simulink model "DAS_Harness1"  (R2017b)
settings: Solver=FixedStepDiscrete  StartTime=0.0  StopTime=1  FixedStep=0.01  RelTol=1e-3  EnableMultiTasking=on
undefined symbols (not defined in the file): sigbuilder_block
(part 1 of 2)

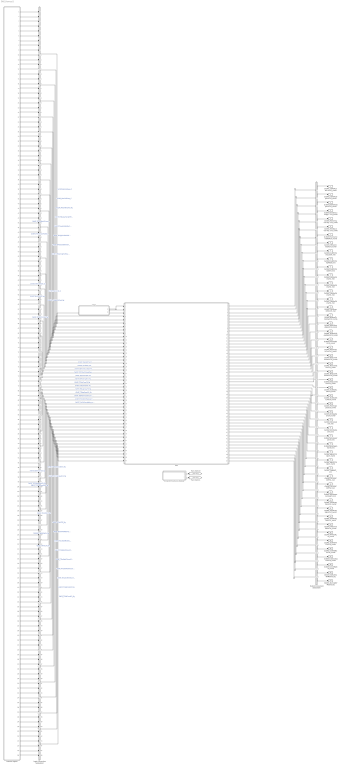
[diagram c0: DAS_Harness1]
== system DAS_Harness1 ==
  Chart : Stateflow chart  TreatAsAtomicUnit=on
  DAS : ModelReference  ModelNameDialog=DAS  SimulationMode=Normal  ModelReferenceVersion='M104C103'
  Harness Inputs : Subsystem  Tag=STV Subsys  LoadFcn=sigbuilder_block('load');  StartFcn=sigbuilder_block('start');  StopFcn=sigbuilder_block('stop');  ClipboardFcn=sigbuilder_block('clipboard');  mask(Sigbuilder block){tuvar=[0:10]}
      mask init:
      | if ~strcmp(get_param(bdroot(gcb),'SimulationStatus'),'stopped'),tuvar = sigbuilder_block('maskInit'); end
  Input Conversion Subsystem : Subsystem  Tag=__SLT_ICS__  Description=Signal spec. and routing
  Output Conversion Subsystem : Subsystem  Tag=__SLT_OCS__  Description=Signal spec. and routing
  Simulink Function scheduler : Test Sequence  Tag=__SLT_FCN_CALL__  TreatAsAtomicUnit=on
  GcDAS_CellVoltLowrLimCnt_numb : Outport  OutDataTypeStr=uint16  PortDimensions=[1]
  GcDAS_CellVoltUpprLimCnt_numb : Outport  Port=2  OutDataTypeStr=uint16  PortDimensions=[1]
  GcDAS_BattVoltUpprLimCnt_numb : Outport  Port=3  OutDataTypeStr=uint16  PortDimensions=[1]
  GcDAS_PackDisCurrUpprLimCnt_numb : Outport  Port=4  OutDataTypeStr=uint16  PortDimensions=[1]
  GcDAS_PackChrgCurrUpprLimCnt_numb : Outport  Port=5  OutDataTypeStr=uint16  PortDimensions=[1]
  GcDAS_FeedbackCurrUpprLimCnt_numb : Outport  Port=6  OutDataTypeStr=uint16  PortDimensions=[1]
  GcDAS_PackCurrLim500ACnt_numb : Outport  Port=7  OutDataTypeStr=uint32  PortDimensions=[1]
  GcDAS_TFPackCrntSafCnt_numb : Outport  Port=8  OutDataTypeStr=uint16  PortDimensions=[1]
  GcDAS_CellMinTempLowTi_min : Outport  Port=9  OutDataTypeStr=single  PortDimensions=[1]
  GcDAS_CellMinTempMidTi_min : Outport  Port=10  OutDataTypeStr=single  PortDimensions=[1]
  GcDAS_CellMinTempHiTi_min : Outport  Port=11  OutDataTypeStr=single  PortDimensions=[1]
  GcDAS_CellMaxTempTi1_min : Outport  Port=12  OutDataTypeStr=single  PortDimensions=[1]
  GcDAS_CellMaxTempTi2_min : Outport  Port=13  OutDataTypeStr=single  PortDimensions=[1]
  GcDAS_CellMaxTempTi3_min : Outport  Port=14  OutDataTypeStr=single  PortDimensions=[1]
  GcDAS_CellMaxTempTi4_min : Outport  Port=15  OutDataTypeStr=single  PortDimensions=[1]
  GcDAS_CellTempDiffLimTi_min : Outport  Port=16  OutDataTypeStr=single  PortDimensions=[1]
  GcDAS_BusbarTempHighCnt_numb : Outport  Port=17  OutDataTypeStr=uint16  PortDimensions=[1]
  GcDAS_PosCtlLoadOpenCnt_numb : Outport  Port=18  OutDataTypeStr=uint16  PortDimensions=[1]
  GcDAS_DCPosCtlLoadOpenCnt_numb : Outport  Port=19  OutDataTypeStr=uint16  PortDimensions=[1]
  GcDAS_PreChrgFailCnt_numb : Outport  Port=20  OutDataTypeStr=uint16  PortDimensions=[1]
  GcDAS_PreChrgOvrCurrCnt_numb : Outport  Port=21  OutDataTypeStr=uint16  PortDimensions=[1]
  GcDAS_PosContAdhesionCnt_numb : Outport  Port=22  OutDataTypeStr=uint16  PortDimensions=[1]
  GcDAS_PosContStuckCnt_numb : Outport  Port=23  OutDataTypeStr=uint16  PortDimensions=[1]
  GcDAS_NegContAdhesionCnt_numb : Outport  Port=24  OutDataTypeStr=uint16  PortDimensions=[1]
  GcDAS_NegContStuckCnt_numb : Outport  Port=25  OutDataTypeStr=uint16  PortDimensions=[1]
  GcDAS_KL30VoltLowCnt_numb : Outport  Port=26  OutDataTypeStr=uint16  PortDimensions=[1]
  GcDAS_KL30CVoltLowCnt_numb : Outport  Port=27  OutDataTypeStr=uint16  PortDimensions=[1]
  GcDAS_PreChrgOpenCnt_numb : Outport  Port=28  OutDataTypeStr=uint16  PortDimensions=[1]
  GcDAS_DCNegOpenCnt_numb : Outport  Port=29  OutDataTypeStr=uint16  PortDimensions=[1]
  GcDAS_SOCLowLimTi_min : Outport  Port=30  OutDataTypeStr=single  PortDimensions=[1]
  GcDAS_SOCHighLimTi_min : Outport  Port=31  OutDataTypeStr=single  PortDimensions=[1]
  GcDAS_SOHLowerLimTi_min : Outport  Port=32  OutDataTypeStr=single  PortDimensions=[1]
  GcDAS_BMSOperationTi_min : Outport  Port=33  OutDataTypeStr=single  PortDimensions=[1]
  GcDAS_BMSACChrgCnt_numb : Outport  Port=34  OutDataTypeStr=uint16  PortDimensions=[1]
  GcDAS_BMSDCChrgCnt_numb : Outport  Port=35  OutDataTypeStr=uint16  PortDimensions=[1]
  GcDAS_CellBalTi_min : Outport  Port=36  OutDataTypeStr=single  PortDimensions=[1]
  GcDAS_OCVSOCDiffTi1_min : Outport  Port=37  OutDataTypeStr=single  PortDimensions=[1]
  GcDAS_OCVSOCDiffTi2_min : Outport  Port=38  OutDataTypeStr=single  PortDimensions=[1]
  GcDAS_SOHLowerLimSaleTi_min : Outport  Port=39  OutDataTypeStr=single  PortDimensions=[1]
  GcDAS_ThmRnwyWarnCnt_numb : Outport  Port=40  OutDataTypeStr=uint16  PortDimensions=[1]
  GcDAS_ThmRnwyAlarmCnt_numb : Outport  Port=41  OutDataTypeStr=uint16  PortDimensions=[1]
  GcDAS_ThmRnwyFaultCnt_numb : Outport  Port=42  OutDataTypeStr=uint16  PortDimensions=[1]
  GcDAS_TPLEventWakeCnt_numb : Outport  Port=43  OutDataTypeStr=uint16  PortDimensions=[1]
  GcDAS_HVILFailCnt_numb : Outport  Port=44  OutDataTypeStr=uint16  PortDimensions=[1]
  GcDAS_IsoHVOFFChkCnt_numb : Outport  Port=45  OutDataTypeStr=uint16  PortDimensions=[1]
  GcDAS_IsoHVONChkCnt_numb : Outport  Port=46  OutDataTypeStr=uint16  PortDimensions=[1]
  GcDAS_IsoDCChrgChkCnt_numb : Outport  Port=47  OutDataTypeStr=uint16  PortDimensions=[1]
  GcDAS_CrashNplCnt_numb : Outport  Port=48  OutDataTypeStr=uint16  PortDimensions=[1]
  GbDAS_HVSafetyNVMStore_flg : Outport  Port=49  OutDataTypeStr=boolean  PortDimensions=[1]
  GbDAS_NormalNVMStore_flg : Outport  Port=50  OutDataTypeStr=boolean  PortDimensions=[1]
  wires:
  Harness Inputs/1(GcCDP_MinCellTemp_C) -> Input Conversion Subsystem/1(Inport_1)
  Harness Inputs/2(GcCDP_MaxCellTemp_C) -> Input Conversion Subsystem/2(Inport_2)
  Harness Inputs/3(GbCDP_AllCellTempVld_flg) -> Input Conversion Subsystem/3(Inport_3)
  Harness Inputs/4(GbISP_TFBusbarTempHiFltLv3_flg) -> Input Conversion Subsystem/4(Inport_4)
  Harness Inputs/5(GbISP_TFLowCellVoltSaf_flg) -> Input Conversion Subsystem/5(Inport_5)
  Harness Inputs/6(GbISP_TFHighCellVoltSaf_flg) -> Input Conversion Subsystem/6(Inport_6)
  Harness Inputs/7(GbISP_TFPackVoltHiAlrmFlt_flg) -> Input Conversion Subsystem/7(Inport_7)
  Harness Inputs/8(GbISP_TFDisChrgPwrFltLevel3_flg) -> Input Conversion Subsystem/8(Inport_8)
  Harness Inputs/9(GbISP_TFChrgPwrFltLevel3_flg) -> Input Conversion Subsystem/9(Inport_9)
  Harness Inputs/10(GbISP_TFFeedbackPwrFltLevel3_flg) -> Input Conversion Subsystem/10(Inport_10)
  Harness Inputs/11(GbISP_TFPackCrntSaf_flg) -> Input Conversion Subsystem/11(Inport_11)
  Harness Inputs/12(GcHDP_PackCrnt_A) -> Input Conversion Subsystem/12(Inport_12)
  Harness Inputs/13(GaCBC_CellBalCtlCmd_flg(1)) -> Input Conversion Subsystem/13(Inport_13)
  Harness Inputs/14(GaCBC_CellBalCtlCmd_flg(2)) -> Input Conversion Subsystem/14(Inport_14)
  Harness Inputs/15(GaCBC_CellBalCtlCmd_flg(3)) -> Input Conversion Subsystem/15(Inport_15)
  Harness Inputs/16(GaCBC_CellBalCtlCmd_flg(4)) -> Input Conversion Subsystem/16(Inport_16)
  Harness Inputs/17(GaCBC_CellBalCtlCmd_flg(5)) -> Input Conversion Subsystem/17(Inport_17)
  Harness Inputs/18(GaCBC_CellBalCtlCmd_flg(6)) -> Input Conversion Subsystem/18(Inport_18)
  Harness Inputs/19(GaCBC_CellBalCtlCmd_flg(7)) -> Input Conversion Subsystem/19(Inport_19)
  Harness Inputs/20(GaCBC_CellBalCtlCmd_flg(8)) -> Input Conversion Subsystem/20(Inport_20)
  Harness Inputs/21(GaCBC_CellBalCtlCmd_flg(9)) -> Input Conversion Subsystem/21(Inport_21)
  Harness Inputs/22(GaCBC_CellBalCtlCmd_flg(10)) -> Input Conversion Subsystem/22(Inport_22)
  Harness Inputs/23(GaCBC_CellBalCtlCmd_flg(11)) -> Input Conversion Subsystem/23(Inport_23)
  Harness Inputs/24(GaCBC_CellBalCtlCmd_flg(12)) -> Input Conversion Subsystem/24(Inport_24)
  Harness Inputs/25(GaCBC_CellBalCtlCmd_flg(13)) -> Input Conversion Subsystem/25(Inport_25)
  Harness Inputs/26(GaCBC_CellBalCtlCmd_flg(14)) -> Input Conversion Subsystem/26(Inport_26)
  Harness Inputs/27(GaCBC_CellBalCtlCmd_flg(15)) -> Input Conversion Subsystem/27(Inport_27)
  Harness Inputs/28(GaCBC_CellBalCtlCmd_flg(16)) -> Input Conversion Subsystem/28(Inport_28)
  Harness Inputs/29(GaCBC_CellBalCtlCmd_flg(17)) -> Input Conversion Subsystem/29(Inport_29)
  Harness Inputs/30(GaCBC_CellBalCtlCmd_flg(18)) -> Input Conversion Subsystem/30(Inport_30)
  Harness Inputs/31(GaCBC_CellBalCtlCmd_flg(19)) -> Input Conversion Subsystem/31(Inport_31)
  Harness Inputs/32(GaCBC_CellBalCtlCmd_flg(20)) -> Input Conversion Subsystem/32(Inport_32)
  Harness Inputs/33(GaCBC_CellBalCtlCmd_flg(21)) -> Input Conversion Subsystem/33(Inport_33)
  Harness Inputs/34(GaCBC_CellBalCtlCmd_flg(22)) -> Input Conversion Subsystem/34(Inport_34)
  Harness Inputs/35(GaCBC_CellBalCtlCmd_flg(23)) -> Input Conversion Subsystem/35(Inport_35)
  Harness Inputs/36(GaCBC_CellBalCtlCmd_flg(24)) -> Input Conversion Subsystem/36(Inport_36)
  Harness Inputs/37(GaCBC_CellBalCtlCmd_flg(25)) -> Input Conversion Subsystem/37(Inport_37)
  Harness Inputs/38(GaCBC_CellBalCtlCmd_flg(26)) -> Input Conversion Subsystem/38(Inport_38)
  Harness Inputs/39(GaCBC_CellBalCtlCmd_flg(27)) -> Input Conversion Subsystem/39(Inport_39)
  Harness Inputs/40(GaCBC_CellBalCtlCmd_flg(28)) -> Input Conversion Subsystem/40(Inport_40)
  Harness Inputs/41(GaCBC_CellBalCtlCmd_flg(29)) -> Input Conversion Subsystem/41(Inport_41)
  Harness Inputs/42(GaCBC_CellBalCtlCmd_flg(30)) -> Input Conversion Subsystem/42(Inport_42)
  Harness Inputs/43(GaCBC_CellBalCtlCmd_flg(31)) -> Input Conversion Subsystem/43(Inport_43)
  Harness Inputs/44(GaCBC_CellBalCtlCmd_flg(32)) -> Input Conversion Subsystem/44(Inport_44)
  Harness Inputs/45(GaCBC_CellBalCtlCmd_flg(33)) -> Input Conversion Subsystem/45(Inport_45)
  Harness Inputs/46(GaCBC_CellBalCtlCmd_flg(34)) -> Input Conversion Subsystem/46(Inport_46)
  Harness Inputs/47(GaCBC_CellBalCtlCmd_flg(35)) -> Input Conversion Subsystem/47(Inport_47)
  Harness Inputs/48(GaCBC_CellBalCtlCmd_flg(36)) -> Input Conversion Subsystem/48(Inport_48)
  Harness Inputs/49(GaCBC_CellBalCtlCmd_flg(37)) -> Input Conversion Subsystem/49(Inport_49)
  Harness Inputs/50(GaCBC_CellBalCtlCmd_flg(38)) -> Input Conversion Subsystem/50(Inport_50)
  Harness Inputs/51(GaCBC_CellBalCtlCmd_flg(39)) -> Input Conversion Subsystem/51(Inport_51)
  Harness Inputs/52(GaCBC_CellBalCtlCmd_flg(40)) -> Input Conversion Subsystem/52(Inport_52)
  Harness Inputs/53(GaCBC_CellBalCtlCmd_flg(41)) -> Input Conversion Subsystem/53(Inport_53)
  Harness Inputs/54(GaCBC_CellBalCtlCmd_flg(42)) -> Input Conversion Subsystem/54(Inport_54)
  Harness Inputs/55(GaCBC_CellBalCtlCmd_flg(43)) -> Input Conversion Subsystem/55(Inport_55)
  Harness Inputs/56(GaCBC_CellBalCtlCmd_flg(44)) -> Input Conversion Subsystem/56(Inport_56)
  Harness Inputs/57(GaCBC_CellBalCtlCmd_flg(45)) -> Input Conversion Subsystem/57(Inport_57)
  Harness Inputs/58(GaCBC_CellBalCtlCmd_flg(46)) -> Input Conversion Subsystem/58(Inport_58)
  Harness Inputs/59(GaCBC_CellBalCtlCmd_flg(47)) -> Input Conversion Subsystem/59(Inport_59)
  Harness Inputs/60(GaCBC_CellBalCtlCmd_flg(48)) -> Input Conversion Subsystem/60(Inport_60)
  Harness Inputs/61(GaCBC_CellBalCtlCmd_flg(49)) -> Input Conversion Subsystem/61(Inport_61)
  Harness Inputs/62(GaCBC_CellBalCtlCmd_flg(50)) -> Input Conversion Subsystem/62(Inport_62)
  Harness Inputs/63(GaCBC_CellBalCtlCmd_flg(51)) -> Input Conversion Subsystem/63(Inport_63)
  Harness Inputs/64(GaCBC_CellBalCtlCmd_flg(52)) -> Input Conversion Subsystem/64(Inport_64)
  Harness Inputs/65(GaCBC_CellBalCtlCmd_flg(53)) -> Input Conversion Subsystem/65(Inport_65)
  Harness Inputs/66(GaCBC_CellBalCtlCmd_flg(54)) -> Input Conversion Subsystem/66(Inport_66)
  Harness Inputs/67(GaCBC_CellBalCtlCmd_flg(55)) -> Input Conversion Subsystem/67(Inport_67)
  Harness Inputs/68(GaCBC_CellBalCtlCmd_flg(56)) -> Input Conversion Subsystem/68(Inport_68)
  Harness Inputs/69(GaCBC_CellBalCtlCmd_flg(57)) -> Input Conversion Subsystem/69(Inport_69)
  Harness Inputs/70(GaCBC_CellBalCtlCmd_flg(58)) -> Input Conversion Subsystem/70(Inport_70)
  Harness Inputs/71(GaCBC_CellBalCtlCmd_flg(59)) -> Input Conversion Subsystem/71(Inport_71)
  Harness Inputs/72(GaCBC_CellBalCtlCmd_flg(60)) -> Input Conversion Subsystem/72(Inport_72)
  Harness Inputs/73(GaCBC_CellBalCtlCmd_flg(61)) -> Input Conversion Subsystem/73(Inport_73)
  Harness Inputs/74(GaCBC_CellBalCtlCmd_flg(62)) -> Input Conversion Subsystem/74(Inport_74)
  Harness Inputs/75(GaCBC_CellBalCtlCmd_flg(63)) -> Input Conversion Subsystem/75(Inport_75)
  Harness Inputs/76(GaCBC_CellBalCtlCmd_flg(64)) -> Input Conversion Subsystem/76(Inport_76)
  Harness Inputs/77(GaCBC_CellBalCtlCmd_flg(65)) -> Input Conversion Subsystem/77(Inport_77)
  Harness Inputs/78(GaCBC_CellBalCtlCmd_flg(66)) -> Input Conversion Subsystem/78(Inport_78)
  Harness Inputs/79(GaCBC_CellBalCtlCmd_flg(67)) -> Input Conversion Subsystem/79(Inport_79)
  Harness Inputs/80(GaCBC_CellBalCtlCmd_flg(68)) -> Input Conversion Subsystem/80(Inport_80)
  Harness Inputs/81(GaCBC_CellBalCtlCmd_flg(69)) -> Input Conversion Subsystem/81(Inport_81)
  Harness Inputs/82(GaCBC_CellBalCtlCmd_flg(70)) -> Input Conversion Subsystem/82(Inport_82)
  Harness Inputs/83(GaCBC_CellBalCtlCmd_flg(71)) -> Input Conversion Subsystem/83(Inport_83)
  Harness Inputs/84(GaCBC_CellBalCtlCmd_flg(72)) -> Input Conversion Subsystem/84(Inport_84)
  Harness Inputs/85(GaCBC_CellBalCtlCmd_flg(73)) -> Input Conversion Subsystem/85(Inport_85)
  Harness Inputs/86(GaCBC_CellBalCtlCmd_flg(74)) -> Input Conversion Subsystem/86(Inport_86)
  Harness Inputs/87(GaCBC_CellBalCtlCmd_flg(75)) -> Input Conversion Subsystem/87(Inport_87)
  Harness Inputs/88(GaCBC_CellBalCtlCmd_flg(76)) -> Input Conversion Subsystem/88(Inport_88)
  Harness Inputs/89(GaCBC_CellBalCtlCmd_flg(77)) -> Input Conversion Subsystem/89(Inport_89)
  Harness Inputs/90(GaCBC_CellBalCtlCmd_flg(78)) -> Input Conversion Subsystem/90(Inport_90)
  Harness Inputs/91(GaCBC_CellBalCtlCmd_flg(79)) -> Input Conversion Subsystem/91(Inport_91)
  Harness Inputs/92(GaCBC_CellBalCtlCmd_flg(80)) -> Input Conversion Subsystem/92(Inport_92)
  Harness Inputs/93(GaCBC_CellBalCtlCmd_flg(81)) -> Input Conversion Subsystem/93(Inport_93)
  Harness Inputs/94(GaCBC_CellBalCtlCmd_flg(82)) -> Input Conversion Subsystem/94(Inport_94)
  Harness Inputs/95(GaCBC_CellBalCtlCmd_flg(83)) -> Input Conversion Subsystem/95(Inport_95)
  Harness Inputs/96(GaCBC_CellBalCtlCmd_flg(84)) -> Input Conversion Subsystem/96(Inport_96)
  Harness Inputs/97(GaCBC_CellBalCtlCmd_flg(85)) -> Input Conversion Subsystem/97(Inport_97)
  Harness Inputs/98(GaCBC_CellBalCtlCmd_flg(86)) -> Input Conversion Subsystem/98(Inport_98)
  Harness Inputs/99(GaCBC_CellBalCtlCmd_flg(87)) -> Input Conversion Subsystem/99(Inport_99)
  Harness Inputs/100(GaCBC_CellBalCtlCmd_flg(88)) -> Input Conversion Subsystem/100(Inport_100)
  Harness Inputs/101(GaCBC_CellBalCtlCmd_flg(89)) -> Input Conversion Subsystem/101(Inport_101)
  Harness Inputs/102(GaCBC_CellBalCtlCmd_flg(90)) -> Input Conversion Subsystem/102(Inport_102)
  Harness Inputs/103(GaCBC_CellBalCtlCmd_flg(91)) -> Input Conversion Subsystem/103(Inport_103)
  Harness Inputs/104(GaCBC_CellBalCtlCmd_flg(92)) -> Input Conversion Subsystem/104(Inport_104)
  Harness Inputs/105(GaCBC_CellBalCtlCmd_flg(93)) -> Input Conversion Subsystem/105(Inport_105)
  Harness Inputs/106(GaCBC_CellBalCtlCmd_flg(94)) -> Input Conversion Subsystem/106(Inport_106)
  Harness Inputs/107(GaCBC_CellBalCtlCmd_flg(95)) -> Input Conversion Subsystem/107(Inport_107)
  Harness Inputs/108(GaCBC_CellBalCtlCmd_flg(96)) -> Input Conversion Subsystem/108(Inport_108)
  Harness Inputs/109(GaCBC_CellBalCtlCmd_flg(97)) -> Input Conversion Subsystem/109(Inport_109)
  Harness Inputs/110(GaCBC_CellBalCtlCmd_flg(98)) -> Input Conversion Subsystem/110(Inport_110)
  Harness Inputs/111(GaCBC_CellBalCtlCmd_flg(99)) -> Input Conversion Subsystem/111(Inport_111)
  Harness Inputs/112(GaCBC_CellBalCtlCmd_flg(100)) -> Input Conversion Subsystem/112(Inport_112)
  Harness Inputs/113(GaCBC_CellBalCtlCmd_flg(101)) -> Input Conversion Subsystem/113(Inport_113)
  Harness Inputs/114(GaCBC_CellBalCtlCmd_flg(102)) -> Input Conversion Subsystem/114(Inport_114)
  Harness Inputs/115(GaCBC_CellBalCtlCmd_flg(103)) -> Input Conversion Subsystem/115(Inport_115)
  Harness Inputs/116(GaCBC_CellBalCtlCmd_flg(104)) -> Input Conversion Subsystem/116(Inport_116)
  Harness Inputs/117(GaCBC_CellBalCtlCmd_flg(105)) -> Input Conversion Subsystem/117(Inport_117)
  Harness Inputs/118(GaCBC_CellBalCtlCmd_flg(106)) -> Input Conversion Subsystem/118(Inport_118)
  Harness Inputs/119(GaCBC_CellBalCtlCmd_flg(107)) -> Input Conversion Subsystem/119(Inport_119)
  Harness Inputs/120(GaCBC_CellBalCtlCmd_flg(108)) -> Input Conversion Subsystem/120(Inport_120)
  Harness Inputs/121(GaCBC_CellBalCtlCmd_flg(109)) -> Input Conversion Subsystem/121(Inport_121)
  Harness Inputs/122(GaCBC_CellBalCtlCmd_flg(110)) -> Input Conversion Subsystem/122(Inport_122)
  Harness Inputs/123(GaCBC_CellBalCtlCmd_flg(111)) -> Input Conversion Subsystem/123(Inport_123)
  Harness Inputs/124(GaCBC_CellBalCtlCmd_flg(112)) -> Input Conversion Subsystem/124(Inport_124)
  Harness Inputs/125(GcSOC_MaxCellSOC_pct) -> Input Conversion Subsystem/125(Inport_125)
  Harness Inputs/126(GcSOC_MinCellSOC_pct) -> Input Conversion Subsystem/126(Inport_126)
  Harness Inputs/127(GcSOC_PackSOC_pct) -> Input Conversion Subsystem/127(Inport_127)
  Harness Inputs/128(GcSOH_PackSOH_pct) -> Input Conversion Subsystem/128(Inport_128)
  Harness Inputs/129(GbISP_TFPosCtlLoadOpenFlt_flg) -> Input Conversion Subsystem/129(Inport_129)
  Harness Inputs/130(GbISP_TFDCPosCtlLoadOpenFlt_flg) -> Input Conversion Subsystem/130(Inport_130)
  Harness Inputs/131(GbISP_TFPreChrgFail_flg) -> Input Conversion Subsystem/131(Inport_131)
  Harness Inputs/132(GbISP_TFPreChrgShrt_flg) -> Input Conversion Subsystem/132(Inport_132)
  Harness Inputs/133(GbISP_TFPosCloseFlt_flg) -> Input Conversion Subsystem/133(Inport_133)
  Harness Inputs/134(GbISP_TFPosOpenFlt_flg) -> Input Conversion Subsystem/134(Inport_134)
  Harness Inputs/135(GbISP_TFNegCloseFlt_flg) -> Input Conversion Subsystem/135(Inport_135)
  Harness Inputs/136(GbISP_TFNegOpenFlt_flg) -> Input Conversion Subsystem/136(Inport_136)
  Harness Inputs/137(GbISP_TFBMUSpyStTooLow_flg) -> Input Conversion Subsystem/137(Inport_137)
  Harness Inputs/138(GbISP_TFKL30CStTooLow_flg) -> Input Conversion Subsystem/138(Inport_138)
  Harness Inputs/139(GeCTC_CtrCtlConnMode_enum) -> Input Conversion Subsystem/139(Inport_139)
  Harness Inputs/140(GbISP_TFPreOpenFlt_flg) -> Input Conversion Subsystem/140(Inport_140)
  Harness Inputs/141(GbISP_TFDCNegOpenFlt_flg) -> Input Conversion Subsystem/141(Inport_141)
  Harness Inputs/142(GbISP_TFThmRnwyWarn_flg) -> Input Conversion Subsystem/142(Inport_142)
  Harness Inputs/143(GbISP_TFThmRnwyAlrm_flg) -> Input Conversion Subsystem/143(Inport_143)
  Harness Inputs/144(GbISP_TFThmRnwyfDet_flg) -> Input Conversion Subsystem/144(Inport_144)
  Harness Inputs/145(GbWSM_TplWkUpPrs_flg) -> Input Conversion Subsystem/145(Inport_145)
  Harness Inputs/146(GbISP_TFHvilLFlt_flg) -> Input Conversion Subsystem/146(Inport_146)
  Harness Inputs/147(GbISP_TFHvilSTG_flg) -> Input Conversion Subsystem/147(Inport_147)
  Harness Inputs/148(GbISP_TFHvilSTV_flg) -> Input Conversion Subsystem/148(Inport_148)
  Harness Inputs/149(GbISP_TFIsoHVoffResFltLevel1_flg) -> Input Conversion Subsystem/149(Inport_149)
  Harness Inputs/150(GbISP_TFIsoHVoffResFltLevel2_flg) -> Input Conversion Subsystem/150(Inport_150)
  Harness Inputs/151(GbISP_TFIsoResFltLevel1_flg) -> Input Conversion Subsystem/151(Inport_151)
  Harness Inputs/152(GbISP_TFIsoResFltLevel2_flg) -> Input Conversion Subsystem/152(Inport_152)
  Harness Inputs/153(GbISP_TFIsoDCResFltLevel1_flg) -> Input Conversion Subsystem/153(Inport_153)
  Harness Inputs/154(GbISP_TFIsoDCResFltLevel2_flg) -> Input Conversion Subsystem/154(Inport_154)
  Harness Inputs/155(GbISP_TFCANCrashFlt_flg) -> Input Conversion Subsystem/155(Inport_155)
  Harness Inputs/156(GbISP_TFHWCrashFlt_flg) -> Input Conversion Subsystem/156(Inport_156)
  Output Conversion Subsystem/1(Outport_1) -> GcDAS_CellVoltLowrLimCnt_numb/1
  Output Conversion Subsystem/2(Outport_2) -> GcDAS_CellVoltUpprLimCnt_numb/1
  Output Conversion Subsystem/3(Outport_3) -> GcDAS_BattVoltUpprLimCnt_numb/1
  Output Conversion Subsystem/4(Outport_4) -> GcDAS_PackDisCurrUpprLimCnt_numb/1
  Output Conversion Subsystem/5(Outport_5) -> GcDAS_PackChrgCurrUpprLimCnt_numb/1
  Output Conversion Subsystem/6(Outport_6) -> GcDAS_FeedbackCurrUpprLimCnt_numb/1
  Output Conversion Subsystem/7(Outport_7) -> GcDAS_PackCurrLim500ACnt_numb/1
  Output Conversion Subsystem/8(Outport_8) -> GcDAS_TFPackCrntSafCnt_numb/1
  Output Conversion Subsystem/9(Outport_9) -> GcDAS_CellMinTempLowTi_min/1
  Output Conversion Subsystem/10(Outport_10) -> GcDAS_CellMinTempMidTi_min/1
  Output Conversion Subsystem/11(Outport_11) -> GcDAS_CellMinTempHiTi_min/1
  Output Conversion Subsystem/12(Outport_12) -> GcDAS_CellMaxTempTi1_min/1
  Output Conversion Subsystem/13(Outport_13) -> GcDAS_CellMaxTempTi2_min/1
  Output Conversion Subsystem/14(Outport_14) -> GcDAS_CellMaxTempTi3_min/1
  Output Conversion Subsystem/15(Outport_15) -> GcDAS_CellMaxTempTi4_min/1
  Output Conversion Subsystem/16(Outport_16) -> GcDAS_CellTempDiffLimTi_min/1
  Output Conversion Subsystem/17(Outport_17) -> GcDAS_BusbarTempHighCnt_numb/1
  Output Conversion Subsystem/18(Outport_18) -> GcDAS_PosCtlLoadOpenCnt_numb/1
  Output Conversion Subsystem/19(Outport_19) -> GcDAS_DCPosCtlLoadOpenCnt_numb/1
  Output Conversion Subsystem/20(Outport_20) -> GcDAS_PreChrgFailCnt_numb/1
  Output Conversion Subsystem/21(Outport_21) -> GcDAS_PreChrgOvrCurrCnt_numb/1
  Output Conversion Subsystem/22(Outport_22) -> GcDAS_PosContAdhesionCnt_numb/1
  Output Conversion Subsystem/23(Outport_23) -> GcDAS_PosContStuckCnt_numb/1
  Output Conversion Subsystem/24(Outport_24) -> GcDAS_NegContAdhesionCnt_numb/1
  Output Conversion Subsystem/25(Outport_25) -> GcDAS_NegContStuckCnt_numb/1
  Output Conversion Subsystem/26(Outport_26) -> GcDAS_KL30VoltLowCnt_numb/1
  Output Conversion Subsystem/27(Outport_27) -> GcDAS_KL30CVoltLowCnt_numb/1
  Output Conversion Subsystem/28(Outport_28) -> GcDAS_PreChrgOpenCnt_numb/1
  Output Conversion Subsystem/29(Outport_29) -> GcDAS_DCNegOpenCnt_numb/1
  Output Conversion Subsystem/30(Outport_30) -> GcDAS_SOCLowLimTi_min/1
  Output Conversion Subsystem/31(Outport_31) -> GcDAS_SOCHighLimTi_min/1
  Output Conversion Subsystem/32(Outport_32) -> GcDAS_SOHLowerLimTi_min/1
  Output Conversion Subsystem/33(Outport_33) -> GcDAS_BMSOperationTi_min/1
  Output Conversion Subsystem/34(Outport_34) -> GcDAS_BMSACChrgCnt_numb/1
  Output Conversion Subsystem/35(Outport_35) -> GcDAS_BMSDCChrgCnt_numb/1
  Output Conversion Subsystem/36(Outport_36) -> GcDAS_CellBalTi_min/1
  Output Conversion Subsystem/37(Outport_37) -> GcDAS_OCVSOCDiffTi1_min/1
  Output Conversion Subsystem/38(Outport_38) -> GcDAS_OCVSOCDiffTi2_min/1
  Output Conversion Subsystem/39(Outport_39) -> GcDAS_SOHLowerLimSaleTi_min/1
  Output Conversion Subsystem/40(Outport_40) -> GcDAS_ThmRnwyWarnCnt_numb/1
  Output Conversion Subsystem/41(Outport_41) -> GcDAS_ThmRnwyAlarmCnt_numb/1
  Output Conversion Subsystem/42(Outport_42) -> GcDAS_ThmRnwyFaultCnt_numb/1
  Output Conversion Subsystem/43(Outport_43) -> GcDAS_TPLEventWakeCnt_numb/1
  Output Conversion Subsystem/44(Outport_44) -> GcDAS_HVILFailCnt_numb/1
  Output Conversion Subsystem/45(Outport_45) -> GcDAS_IsoHVOFFChkCnt_numb/1
  Output Conversion Subsystem/46(Outport_46) -> GcDAS_IsoHVONChkCnt_numb/1
  Output Conversion Subsystem/47(Outport_47) -> GcDAS_IsoDCChrgChkCnt_numb/1
  Output Conversion Subsystem/48(Outport_48) -> GcDAS_CrashNplCnt_numb/1
  Output Conversion Subsystem/49(Outport_49) -> GbDAS_HVSafetyNVMStore_flg/1
  Output Conversion Subsystem/50(Outport_50) -> GbDAS_NormalNVMStore_flg/1
  Input Conversion Subsystem/3(Outport_3) -> DAS/3  "GcCDP_MinCellTemp_C"
  Input Conversion Subsystem/4(Outport_4) -> DAS/4  "GcCDP_MaxCellTemp_C"
  Input Conversion Subsystem/5(Outport_5) -> DAS/5  "GbCDP_AllCellTempVld_flg"
  Input Conversion Subsystem/6(Outport_6) -> DAS/6  "GbISP_TFBusbarTempHiFltLv3_flg"
  Input Conversion Subsystem/7(Outport_7) -> DAS/7  "GbISP_TFLowCellVoltSaf_flg"
  Input Conversion Subsystem/8(Outport_8) -> DAS/8  "GbISP_TFHighCellVoltSaf_flg"
  Input Conversion Subsystem/9(Outport_9) -> DAS/9  "GbISP_TFPackVoltHiAlrmFlt_flg"
  Input Conversion Subsystem/10(Outport_10) -> DAS/10  "GbISP_TFDisChrgPwrFltLevel3_flg"
  Input Conversion Subsystem/11(Outport_11) -> DAS/11  "GbISP_TFChrgPwrFltLevel3_flg"
  Input Conversion Subsystem/12(Outport_12) -> DAS/12  "GbISP_TFFeedbackPwrFltLevel3_flg"
  Input Conversion Subsystem/13(Outport_13) -> DAS/13  "GbISP_TFPackCrntSaf_flg"
  Input Conversion Subsystem/14(Outport_14) -> DAS/14  "GcHDP_PackCrnt_A"
  Input Conversion Subsystem/15(Outport_15) -> DAS/15  "GaCBC_CellBalCtlCmd_flg"
  Input Conversion Subsystem/16(Outport_16) -> DAS/16  "GcSOC_MaxCellSOC_pct"
  Input Conversion Subsystem/17(Outport_17) -> DAS/17  "GcSOC_MinCellSOC_pct"
  Input Conversion Subsystem/18(Outport_18) -> DAS/18  "GcSOC_PackSOC_pct"
  Input Conversion Subsystem/19(Outport_19) -> DAS/19  "GcSOH_PackSOH_pct"
  Input Conversion Subsystem/20(Outport_20) -> DAS/20  "GbISP_TFPosCtlLoadOpenFlt_flg"
  Input Conversion Subsystem/21(Outport_21) -> DAS/21  "GbISP_TFDCPosCtlLoadOpenFlt_flg"
  Input Conversion Subsystem/22(Outport_22) -> DAS/22  "GbISP_TFPreChrgFail_flg"
  Input Conversion Subsystem/23(Outport_23) -> DAS/23  "GbISP_TFPreChrgShrt_flg"
  Input Conversion Subsystem/24(Outport_24) -> DAS/24  "GbISP_TFPosCloseFlt_flg"
  Input Conversion Subsystem/25(Outport_25) -> DAS/25  "GbISP_TFPosOpenFlt_flg"
  Input Conversion Subsystem/26(Outport_26) -> DAS/26  "GbISP_TFNegCloseFlt_flg"
  Input Conversion Subsystem/27(Outport_27) -> DAS/27  "GbISP_TFNegOpenFlt_flg"
  Input Conversion Subsystem/28(Outport_28) -> DAS/28  "GbISP_TFBMUSpyStTooLow_flg"
  Input Conversion Subsystem/29(Outport_29) -> DAS/29  "GbISP_TFKL30CStTooLow_flg"
  Input Conversion Subsystem/30(Outport_30) -> DAS/30  "GeCTC_CtrCtlConnMode_enum"
  Input Conversion Subsystem/31(Outport_31) -> DAS/31  "GbISP_TFPreOpenFlt_flg"
  Input Conversion Subsystem/32(Outport_32) -> DAS/32  "GbISP_TFDCNegOpenFlt_flg"
  Input Conversion Subsystem/33(Outport_33) -> DAS/33  "GbISP_TFThmRnwyWarn_flg"
  Input Conversion Subsystem/34(Outport_34) -> DAS/34  "GbISP_TFThmRnwyAlrm_flg"
  Input Conversion Subsystem/35(Outport_35) -> DAS/35  "GbISP_TFThmRnwyfDet_flg"
  Input Conversion Subsystem/36(Outport_36) -> DAS/36  "GbWSM_TplWkUpPrs_flg"
  Input Conversion Subsystem/37(Outport_37) -> DAS/37  "GbISP_TFHvilLFlt_flg"
  Input Conversion Subsystem/38(Outport_38) -> DAS/38  "GbISP_TFHvilSTG_flg"
  Input Conversion Subsystem/39(Outport_39) -> DAS/39  "GbISP_TFHvilSTV_flg"
  Input Conversion Subsystem/40(Outport_40) -> DAS/40  "GbISP_TFIsoHVoffResFltLevel1_flg"
  Input Conversion Subsystem/41(Outport_41) -> DAS/41  "GbISP_TFIsoHVoffResFltLevel2_flg"
  Input Conversion Subsystem/42(Outport_42) -> DAS/42  "GbISP_TFIsoResFltLevel1_flg"
  Input Conversion Subsystem/43(Outport_43) -> DAS/43  "GbISP_TFIsoResFltLevel2_flg"
  Input Conversion Subsystem/44(Outport_44) -> DAS/44  "GbISP_TFIsoDCResFltLevel1_flg"
  Input Conversion Subsystem/45(Outport_45) -> DAS/45  "GbISP_TFIsoDCResFltLevel2_flg"
  Input Conversion Subsystem/46(Outport_46) -> DAS/46  "GbISP_TFCANCrashFlt_flg"
  Input Conversion Subsystem/47(Outport_47) -> DAS/47  "GbISP_TFHWCrashFlt_flg"
  DAS/1 -> Output Conversion Subsystem/1(Inport_1)
  DAS/2 -> Output Conversion Subsystem/2(Inport_2)
  DAS/3 -> Output Conversion Subsystem/3(Inport_3)
  DAS/4 -> Output Conversion Subsystem/4(Inport_4)
  DAS/5 -> Output Conversion Subsystem/5(Inport_5)
  DAS/6 -> Output Conversion Subsystem/6(Inport_6)
  DAS/7 -> Output Conversion Subsystem/7(Inport_7)
  DAS/8 -> Output Conversion Subsystem/8(Inport_8)
  DAS/9 -> Output Conversion Subsystem/9(Inport_9)
  DAS/10 -> Output Conversion Subsystem/10(Inport_10)
  DAS/11 -> Output Conversion Subsystem/11(Inport_11)
  DAS/12 -> Output Conversion Subsystem/12(Inport_12)
  DAS/13 -> Output Conversion Subsystem/13(Inport_13)
  DAS/14 -> Output Conversion Subsystem/14(Inport_14)
  DAS/15 -> Output Conversion Subsystem/15(Inport_15)
  DAS/16 -> Output Conversion Subsystem/16(Inport_16)
  DAS/17 -> Output Conversion Subsystem/17(Inport_17)
  DAS/18 -> Output Conversion Subsystem/18(Inport_18)
  DAS/19 -> Output Conversion Subsystem/19(Inport_19)
  DAS/20 -> Output Conversion Subsystem/20(Inport_20)
  DAS/21 -> Output Conversion Subsystem/21(Inport_21)
  DAS/22 -> Output Conversion Subsystem/22(Inport_22)
  DAS/23 -> Output Conversion Subsystem/23(Inport_23)
  DAS/24 -> Output Conversion Subsystem/24(Inport_24)
  DAS/25 -> Output Conversion Subsystem/25(Inport_25)
  DAS/26 -> Output Conversion Subsystem/26(Inport_26)
  DAS/27 -> Output Conversion Subsystem/27(Inport_27)
  DAS/28 -> Output Conversion Subsystem/28(Inport_28)
  DAS/29 -> Output Conversion Subsystem/29(Inport_29)
  DAS/30 -> Output Conversion Subsystem/30(Inport_30)
  DAS/31 -> Output Conversion Subsystem/31(Inport_31)
  DAS/32 -> Output Conversion Subsystem/32(Inport_32)
  DAS/33 -> Output Conversion Subsystem/33(Inport_33)
  DAS/34 -> Output Conversion Subsystem/34(Inport_34)
  DAS/35 -> Output Conversion Subsystem/35(Inport_35)
  DAS/36 -> Output Conversion Subsystem/36(Inport_36)
  DAS/37 -> Output Conversion Subsystem/37(Inport_37)
  DAS/38 -> Output Conversion Subsystem/38(Inport_38)
  DAS/39 -> Output Conversion Subsystem/39(Inport_39)
  DAS/40 -> Output Conversion Subsystem/40(Inport_40)
  DAS/41 -> Output Conversion Subsystem/41(Inport_41)
  DAS/42 -> Output Conversion Subsystem/42(Inport_42)
  DAS/43 -> Output Conversion Subsystem/43(Inport_43)
  DAS/44 -> Output Conversion Subsystem/44(Inport_44)
  DAS/45 -> Output Conversion Subsystem/45(Inport_45)
  DAS/46 -> Output Conversion Subsystem/46(Inport_46)
  DAS/47 -> Output Conversion Subsystem/47(Inport_47)
  DAS/48 -> Output Conversion Subsystem/48(Inport_48)
  DAS/49 -> Output Conversion Subsystem/49(Inport_49)
  DAS/50 -> Output Conversion Subsystem/50(Inport_50)
  Simulink Function scheduler/1(DAS_DataFastAbsStr_10ms()) -> [send_fcn1]
  Simulink Function scheduler/2(DAS_DataSlowAbsStr_100ms()) -> [send_fcn2]
  Chart/2(Run100ms()) -> DAS/2
  Chart/1(Run10ms()) -> DAS/1

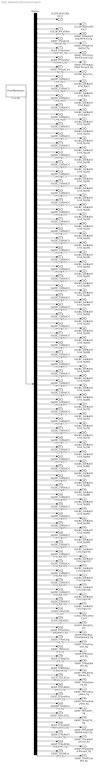
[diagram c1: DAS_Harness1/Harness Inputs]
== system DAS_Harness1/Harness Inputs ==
  Demux : Demux  Tag=STV Demux  Outputs=156
  FromWs : FromWorkspace  Tag=STV FromWs  VariableName=tuvar  SampleTime=0
  GcCDP_MinCellTemp_C : Outport  Tag=STV Outport
  GcCDP_MaxCellTemp_C : Outport  Tag=STV Outport  Port=2
  GbCDP_AllCellTempVld_flg : Outport  Tag=STV Outport  Port=3
  GbISP_TFBusbarTempHiFltLv3_flg : Outport  Tag=STV Outport  Port=4
  GbISP_TFLowCellVoltSaf_flg : Outport  Tag=STV Outport  Port=5
  GbISP_TFHighCellVoltSaf_flg : Outport  Tag=STV Outport  Port=6
  GbISP_TFPackVoltHiAlrmFlt_flg : Outport  Tag=STV Outport  Port=7
  GbISP_TFDisChrgPwrFltLevel3_flg : Outport  Tag=STV Outport  Port=8
  GbISP_TFChrgPwrFltLevel3_flg : Outport  Tag=STV Outport  Port=9
  GbISP_TFFeedbackPwrFltLevel3_flg : Outport  Tag=STV Outport  Port=10
  GbISP_TFPackCrntSaf_flg : Outport  Tag=STV Outport  Port=11
  GcHDP_PackCrnt_A : Outport  Tag=STV Outport  Port=12
  GaCBC_CellBalCtlCmd_flg(1) : Outport  Tag=STV Outport  Port=13
  GaCBC_CellBalCtlCmd_flg(2) : Outport  Tag=STV Outport  Port=14
  GaCBC_CellBalCtlCmd_flg(3) : Outport  Tag=STV Outport  Port=15
  GaCBC_CellBalCtlCmd_flg(4) : Outport  Tag=STV Outport  Port=16
  GaCBC_CellBalCtlCmd_flg(5) : Outport  Tag=STV Outport  Port=17
  GaCBC_CellBalCtlCmd_flg(6) : Outport  Tag=STV Outport  Port=18
  GaCBC_CellBalCtlCmd_flg(7) : Outport  Tag=STV Outport  Port=19
  GaCBC_CellBalCtlCmd_flg(8) : Outport  Tag=STV Outport  Port=20
  GaCBC_CellBalCtlCmd_flg(9) : Outport  Tag=STV Outport  Port=21
  GaCBC_CellBalCtlCmd_flg(10) : Outport  Tag=STV Outport  Port=22
  GaCBC_CellBalCtlCmd_flg(11) : Outport  Tag=STV Outport  Port=23
  GaCBC_CellBalCtlCmd_flg(12) : Outport  Tag=STV Outport  Port=24
  GaCBC_CellBalCtlCmd_flg(13) : Outport  Tag=STV Outport  Port=25
  GaCBC_CellBalCtlCmd_flg(14) : Outport  Tag=STV Outport  Port=26
  GaCBC_CellBalCtlCmd_flg(15) : Outport  Tag=STV Outport  Port=27
  GaCBC_CellBalCtlCmd_flg(16) : Outport  Tag=STV Outport  Port=28
  GaCBC_CellBalCtlCmd_flg(17) : Outport  Tag=STV Outport  Port=29
  GaCBC_CellBalCtlCmd_flg(18) : Outport  Tag=STV Outport  Port=30
  GaCBC_CellBalCtlCmd_flg(19) : Outport  Tag=STV Outport  Port=31
  GaCBC_CellBalCtlCmd_flg(20) : Outport  Tag=STV Outport  Port=32
  GaCBC_CellBalCtlCmd_flg(21) : Outport  Tag=STV Outport  Port=33
  GaCBC_CellBalCtlCmd_flg(22) : Outport  Tag=STV Outport  Port=34
  GaCBC_CellBalCtlCmd_flg(23) : Outport  Tag=STV Outport  Port=35
  GaCBC_CellBalCtlCmd_flg(24) : Outport  Tag=STV Outport  Port=36
  GaCBC_CellBalCtlCmd_flg(25) : Outport  Tag=STV Outport  Port=37
  GaCBC_CellBalCtlCmd_flg(26) : Outport  Tag=STV Outport  Port=38
  GaCBC_CellBalCtlCmd_flg(27) : Outport  Tag=STV Outport  Port=39
  GaCBC_CellBalCtlCmd_flg(28) : Outport  Tag=STV Outport  Port=40
  GaCBC_CellBalCtlCmd_flg(29) : Outport  Tag=STV Outport  Port=41
  GaCBC_CellBalCtlCmd_flg(30) : Outport  Tag=STV Outport  Port=42
  GaCBC_CellBalCtlCmd_flg(31) : Outport  Tag=STV Outport  Port=43
  GaCBC_CellBalCtlCmd_flg(32) : Outport  Tag=STV Outport  Port=44
  GaCBC_CellBalCtlCmd_flg(33) : Outport  Tag=STV Outport  Port=45
  GaCBC_CellBalCtlCmd_flg(34) : Outport  Tag=STV Outport  Port=46
  GaCBC_CellBalCtlCmd_flg(35) : Outport  Tag=STV Outport  Port=47
  GaCBC_CellBalCtlCmd_flg(36) : Outport  Tag=STV Outport  Port=48
  GaCBC_CellBalCtlCmd_flg(37) : Outport  Tag=STV Outport  Port=49
  GaCBC_CellBalCtlCmd_flg(38) : Outport  Tag=STV Outport  Port=50
  GaCBC_CellBalCtlCmd_flg(39) : Outport  Tag=STV Outport  Port=51
  GaCBC_CellBalCtlCmd_flg(40) : Outport  Tag=STV Outport  Port=52
  GaCBC_CellBalCtlCmd_flg(41) : Outport  Tag=STV Outport  Port=53
  GaCBC_CellBalCtlCmd_flg(42) : Outport  Tag=STV Outport  Port=54
  GaCBC_CellBalCtlCmd_flg(43) : Outport  Tag=STV Outport  Port=55
  GaCBC_CellBalCtlCmd_flg(44) : Outport  Tag=STV Outport  Port=56
  GaCBC_CellBalCtlCmd_flg(45) : Outport  Tag=STV Outport  Port=57
  GaCBC_CellBalCtlCmd_flg(46) : Outport  Tag=STV Outport  Port=58
  GaCBC_CellBalCtlCmd_flg(47) : Outport  Tag=STV Outport  Port=59
  GaCBC_CellBalCtlCmd_flg(48) : Outport  Tag=STV Outport  Port=60
  GaCBC_CellBalCtlCmd_flg(49) : Outport  Tag=STV Outport  Port=61
  GaCBC_CellBalCtlCmd_flg(50) : Outport  Tag=STV Outport  Port=62
  GaCBC_CellBalCtlCmd_flg(51) : Outport  Tag=STV Outport  Port=63
  GaCBC_CellBalCtlCmd_flg(52) : Outport  Tag=STV Outport  Port=64
  GaCBC_CellBalCtlCmd_flg(53) : Outport  Tag=STV Outport  Port=65
  GaCBC_CellBalCtlCmd_flg(54) : Outport  Tag=STV Outport  Port=66
  GaCBC_CellBalCtlCmd_flg(55) : Outport  Tag=STV Outport  Port=67
  GaCBC_CellBalCtlCmd_flg(56) : Outport  Tag=STV Outport  Port=68
  GaCBC_CellBalCtlCmd_flg(57) : Outport  Tag=STV Outport  Port=69
  GaCBC_CellBalCtlCmd_flg(58) : Outport  Tag=STV Outport  Port=70
  GaCBC_CellBalCtlCmd_flg(59) : Outport  Tag=STV Outport  Port=71
  GaCBC_CellBalCtlCmd_flg(60) : Outport  Tag=STV Outport  Port=72
  GaCBC_CellBalCtlCmd_flg(61) : Outport  Tag=STV Outport  Port=73
  GaCBC_CellBalCtlCmd_flg(62) : Outport  Tag=STV Outport  Port=74
  GaCBC_CellBalCtlCmd_flg(63) : Outport  Tag=STV Outport  Port=75
  GaCBC_CellBalCtlCmd_flg(64) : Outport  Tag=STV Outport  Port=76
  GaCBC_CellBalCtlCmd_flg(65) : Outport  Tag=STV Outport  Port=77
  GaCBC_CellBalCtlCmd_flg(66) : Outport  Tag=STV Outport  Port=78
  GaCBC_CellBalCtlCmd_flg(67) : Outport  Tag=STV Outport  Port=79
  GaCBC_CellBalCtlCmd_flg(68) : Outport  Tag=STV Outport  Port=80
  GaCBC_CellBalCtlCmd_flg(69) : Outport  Tag=STV Outport  Port=81
  GaCBC_CellBalCtlCmd_flg(70) : Outport  Tag=STV Outport  Port=82
  GaCBC_CellBalCtlCmd_flg(71) : Outport  Tag=STV Outport  Port=83
  GaCBC_CellBalCtlCmd_flg(72) : Outport  Tag=STV Outport  Port=84
  GaCBC_CellBalCtlCmd_flg(73) : Outport  Tag=STV Outport  Port=85
  GaCBC_CellBalCtlCmd_flg(74) : Outport  Tag=STV Outport  Port=86
  GaCBC_CellBalCtlCmd_flg(75) : Outport  Tag=STV Outport  Port=87
  GaCBC_CellBalCtlCmd_flg(76) : Outport  Tag=STV Outport  Port=88
  GaCBC_CellBalCtlCmd_flg(77) : Outport  Tag=STV Outport  Port=89
  GaCBC_CellBalCtlCmd_flg(78) : Outport  Tag=STV Outport  Port=90
  GaCBC_CellBalCtlCmd_flg(79) : Outport  Tag=STV Outport  Port=91
  GaCBC_CellBalCtlCmd_flg(80) : Outport  Tag=STV Outport  Port=92
  GaCBC_CellBalCtlCmd_flg(81) : Outport  Tag=STV Outport  Port=93
  GaCBC_CellBalCtlCmd_flg(82) : Outport  Tag=STV Outport  Port=94
  GaCBC_CellBalCtlCmd_flg(83) : Outport  Tag=STV Outport  Port=95
  GaCBC_CellBalCtlCmd_flg(84) : Outport  Tag=STV Outport  Port=96
  GaCBC_CellBalCtlCmd_flg(85) : Outport  Tag=STV Outport  Port=97
  GaCBC_CellBalCtlCmd_flg(86) : Outport  Tag=STV Outport  Port=98
  GaCBC_CellBalCtlCmd_flg(87) : Outport  Tag=STV Outport  Port=99
  GaCBC_CellBalCtlCmd_flg(88) : Outport  Tag=STV Outport  Port=100
  GaCBC_CellBalCtlCmd_flg(89) : Outport  Tag=STV Outport  Port=101
  GaCBC_CellBalCtlCmd_flg(90) : Outport  Tag=STV Outport  Port=102
  GaCBC_CellBalCtlCmd_flg(91) : Outport  Tag=STV Outport  Port=103
  GaCBC_CellBalCtlCmd_flg(92) : Outport  Tag=STV Outport  Port=104
  GaCBC_CellBalCtlCmd_flg(93) : Outport  Tag=STV Outport  Port=105
  GaCBC_CellBalCtlCmd_flg(94) : Outport  Tag=STV Outport  Port=106
  GaCBC_CellBalCtlCmd_flg(95) : Outport  Tag=STV Outport  Port=107
  GaCBC_CellBalCtlCmd_flg(96) : Outport  Tag=STV Outport  Port=108
  GaCBC_CellBalCtlCmd_flg(97) : Outport  Tag=STV Outport  Port=109
  GaCBC_CellBalCtlCmd_flg(98) : Outport  Tag=STV Outport  Port=110
  GaCBC_CellBalCtlCmd_flg(99) : Outport  Tag=STV Outport  Port=111
  GaCBC_CellBalCtlCmd_flg(100) : Outport  Tag=STV Outport  Port=112
  GaCBC_CellBalCtlCmd_flg(101) : Outport  Tag=STV Outport  Port=113
  GaCBC_CellBalCtlCmd_flg(102) : Outport  Tag=STV Outport  Port=114
  GaCBC_CellBalCtlCmd_flg(103) : Outport  Tag=STV Outport  Port=115
  GaCBC_CellBalCtlCmd_flg(104) : Outport  Tag=STV Outport  Port=116
  GaCBC_CellBalCtlCmd_flg(105) : Outport  Tag=STV Outport  Port=117
  GaCBC_CellBalCtlCmd_flg(106) : Outport  Tag=STV Outport  Port=118
  GaCBC_CellBalCtlCmd_flg(107) : Outport  Tag=STV Outport  Port=119
  GaCBC_CellBalCtlCmd_flg(108) : Outport  Tag=STV Outport  Port=120
  GaCBC_CellBalCtlCmd_flg(109) : Outport  Tag=STV Outport  Port=121
  GaCBC_CellBalCtlCmd_flg(110) : Outport  Tag=STV Outport  Port=122
  GaCBC_CellBalCtlCmd_flg(111) : Outport  Tag=STV Outport  Port=123
  GaCBC_CellBalCtlCmd_flg(112) : Outport  Tag=STV Outport  Port=124
  GcSOC_MaxCellSOC_pct : Outport  Tag=STV Outport  Port=125
  GcSOC_MinCellSOC_pct : Outport  Tag=STV Outport  Port=126
  GcSOC_PackSOC_pct : Outport  Tag=STV Outport  Port=127
  GcSOH_PackSOH_pct : Outport  Tag=STV Outport  Port=128
  GbISP_TFPosCtlLoadOpenFlt_flg : Outport  Tag=STV Outport  Port=129
  GbISP_TFDCPosCtlLoadOpenFlt_flg : Outport  Tag=STV Outport  Port=130
  GbISP_TFPreChrgFail_flg : Outport  Tag=STV Outport  Port=131
  GbISP_TFPreChrgShrt_flg : Outport  Tag=STV Outport  Port=132
  GbISP_TFPosCloseFlt_flg : Outport  Tag=STV Outport  Port=133
  GbISP_TFPosOpenFlt_flg : Outport  Tag=STV Outport  Port=134
  GbISP_TFNegCloseFlt_flg : Outport  Tag=STV Outport  Port=135
  GbISP_TFNegOpenFlt_flg : Outport  Tag=STV Outport  Port=136
  GbISP_TFBMUSpyStTooLow_flg : Outport  Tag=STV Outport  Port=137
  GbISP_TFKL30CStTooLow_flg : Outport  Tag=STV Outport  Port=138
  GeCTC_CtrCtlConnMode_enum : Outport  Tag=STV Outport  Port=139
  GbISP_TFPreOpenFlt_flg : Outport  Tag=STV Outport  Port=140
  GbISP_TFDCNegOpenFlt_flg : Outport  Tag=STV Outport  Port=141
  GbISP_TFThmRnwyWarn_flg : Outport  Tag=STV Outport  Port=142
  GbISP_TFThmRnwyAlrm_flg : Outport  Tag=STV Outport  Port=143
  GbISP_TFThmRnwyfDet_flg : Outport  Tag=STV Outport  Port=144
  GbWSM_TplWkUpPrs_flg : Outport  Tag=STV Outport  Port=145
  GbISP_TFHvilLFlt_flg : Outport  Tag=STV Outport  Port=146
  GbISP_TFHvilSTG_flg : Outport  Tag=STV Outport  Port=147
  GbISP_TFHvilSTV_flg : Outport  Tag=STV Outport  Port=148
  GbISP_TFIsoHVoffResFltLevel1_flg : Outport  Tag=STV Outport  Port=149
  GbISP_TFIsoHVoffResFltLevel2_flg : Outport  Tag=STV Outport  Port=150
  GbISP_TFIsoResFltLevel1_flg : Outport  Tag=STV Outport  Port=151
  GbISP_TFIsoResFltLevel2_flg : Outport  Tag=STV Outport  Port=152
  GbISP_TFIsoDCResFltLevel1_flg : Outport  Tag=STV Outport  Port=153
  GbISP_TFIsoDCResFltLevel2_flg : Outport  Tag=STV Outport  Port=154
  GbISP_TFCANCrashFlt_flg : Outport  Tag=STV Outport  Port=155
  GbISP_TFHWCrashFlt_flg : Outport  Tag=STV Outport  Port=156
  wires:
  FromWs/1 -> Demux/1
  Demux/1 -> GcCDP_MinCellTemp_C/1
  Demux/2 -> GcCDP_MaxCellTemp_C/1
  Demux/3 -> GbCDP_AllCellTempVld_flg/1
  Demux/4 -> GbISP_TFBusbarTempHiFltLv3_flg/1
  Demux/5 -> GbISP_TFLowCellVoltSaf_flg/1
  Demux/6 -> GbISP_TFHighCellVoltSaf_flg/1
  Demux/7 -> GbISP_TFPackVoltHiAlrmFlt_flg/1
  Demux/8 -> GbISP_TFDisChrgPwrFltLevel3_flg/1
  Demux/9 -> GbISP_TFChrgPwrFltLevel3_flg/1
  Demux/10 -> GbISP_TFFeedbackPwrFltLevel3_flg/1
  Demux/11 -> GbISP_TFPackCrntSaf_flg/1
  Demux/12 -> GcHDP_PackCrnt_A/1
  Demux/13 -> GaCBC_CellBalCtlCmd_flg(1)/1
  Demux/14 -> GaCBC_CellBalCtlCmd_flg(2)/1
  Demux/15 -> GaCBC_CellBalCtlCmd_flg(3)/1
  Demux/16 -> GaCBC_CellBalCtlCmd_flg(4)/1
  Demux/17 -> GaCBC_CellBalCtlCmd_flg(5)/1
  Demux/18 -> GaCBC_CellBalCtlCmd_flg(6)/1
  Demux/19 -> GaCBC_CellBalCtlCmd_flg(7)/1
  Demux/20 -> GaCBC_CellBalCtlCmd_flg(8)/1
  Demux/21 -> GaCBC_CellBalCtlCmd_flg(9)/1
  Demux/22 -> GaCBC_CellBalCtlCmd_flg(10)/1
  Demux/23 -> GaCBC_CellBalCtlCmd_flg(11)/1
  Demux/24 -> GaCBC_CellBalCtlCmd_flg(12)/1
  Demux/25 -> GaCBC_CellBalCtlCmd_flg(13)/1
  Demux/26 -> GaCBC_CellBalCtlCmd_flg(14)/1
  Demux/27 -> GaCBC_CellBalCtlCmd_flg(15)/1
  Demux/28 -> GaCBC_CellBalCtlCmd_flg(16)/1
  Demux/29 -> GaCBC_CellBalCtlCmd_flg(17)/1
  Demux/30 -> GaCBC_CellBalCtlCmd_flg(18)/1
  Demux/31 -> GaCBC_CellBalCtlCmd_flg(19)/1
  Demux/32 -> GaCBC_CellBalCtlCmd_flg(20)/1
  Demux/33 -> GaCBC_CellBalCtlCmd_flg(21)/1
  Demux/34 -> GaCBC_CellBalCtlCmd_flg(22)/1
  Demux/35 -> GaCBC_CellBalCtlCmd_flg(23)/1
  Demux/36 -> GaCBC_CellBalCtlCmd_flg(24)/1
  Demux/37 -> GaCBC_CellBalCtlCmd_flg(25)/1
  Demux/38 -> GaCBC_CellBalCtlCmd_flg(26)/1
  Demux/39 -> GaCBC_CellBalCtlCmd_flg(27)/1
  Demux/40 -> GaCBC_CellBalCtlCmd_flg(28)/1
  Demux/41 -> GaCBC_CellBalCtlCmd_flg(29)/1
  Demux/42 -> GaCBC_CellBalCtlCmd_flg(30)/1
  Demux/43 -> GaCBC_CellBalCtlCmd_flg(31)/1
  Demux/44 -> GaCBC_CellBalCtlCmd_flg(32)/1
  Demux/45 -> GaCBC_CellBalCtlCmd_flg(33)/1
  Demux/46 -> GaCBC_CellBalCtlCmd_flg(34)/1
  Demux/47 -> GaCBC_CellBalCtlCmd_flg(35)/1
  Demux/48 -> GaCBC_CellBalCtlCmd_flg(36)/1
  Demux/49 -> GaCBC_CellBalCtlCmd_flg(37)/1
  Demux/50 -> GaCBC_CellBalCtlCmd_flg(38)/1
  Demux/51 -> GaCBC_CellBalCtlCmd_flg(39)/1
  Demux/52 -> GaCBC_CellBalCtlCmd_flg(40)/1
  Demux/53 -> GaCBC_CellBalCtlCmd_flg(41)/1
  Demux/54 -> GaCBC_CellBalCtlCmd_flg(42)/1
  Demux/55 -> GaCBC_CellBalCtlCmd_flg(43)/1
  Demux/56 -> GaCBC_CellBalCtlCmd_flg(44)/1
  Demux/57 -> GaCBC_CellBalCtlCmd_flg(45)/1
  Demux/58 -> GaCBC_CellBalCtlCmd_flg(46)/1
  Demux/59 -> GaCBC_CellBalCtlCmd_flg(47)/1
  Demux/60 -> GaCBC_CellBalCtlCmd_flg(48)/1
  Demux/61 -> GaCBC_CellBalCtlCmd_flg(49)/1
  Demux/62 -> GaCBC_CellBalCtlCmd_flg(50)/1
  Demux/63 -> GaCBC_CellBalCtlCmd_flg(51)/1
  Demux/64 -> GaCBC_CellBalCtlCmd_flg(52)/1
  Demux/65 -> GaCBC_CellBalCtlCmd_flg(53)/1
  Demux/66 -> GaCBC_CellBalCtlCmd_flg(54)/1
  Demux/67 -> GaCBC_CellBalCtlCmd_flg(55)/1
  Demux/68 -> GaCBC_CellBalCtlCmd_flg(56)/1
  Demux/69 -> GaCBC_CellBalCtlCmd_flg(57)/1
  Demux/70 -> GaCBC_CellBalCtlCmd_flg(58)/1
  Demux/71 -> GaCBC_CellBalCtlCmd_flg(59)/1
  Demux/72 -> GaCBC_CellBalCtlCmd_flg(60)/1
  Demux/73 -> GaCBC_CellBalCtlCmd_flg(61)/1
  Demux/74 -> GaCBC_CellBalCtlCmd_flg(62)/1
  Demux/75 -> GaCBC_CellBalCtlCmd_flg(63)/1
  Demux/76 -> GaCBC_CellBalCtlCmd_flg(64)/1
  Demux/77 -> GaCBC_CellBalCtlCmd_flg(65)/1
  Demux/78 -> GaCBC_CellBalCtlCmd_flg(66)/1
  Demux/79 -> GaCBC_CellBalCtlCmd_flg(67)/1
  Demux/80 -> GaCBC_CellBalCtlCmd_flg(68)/1
  Demux/81 -> GaCBC_CellBalCtlCmd_flg(69)/1
  Demux/82 -> GaCBC_CellBalCtlCmd_flg(70)/1
  Demux/83 -> GaCBC_CellBalCtlCmd_flg(71)/1
  Demux/84 -> GaCBC_CellBalCtlCmd_flg(72)/1
  Demux/85 -> GaCBC_CellBalCtlCmd_flg(73)/1
  Demux/86 -> GaCBC_CellBalCtlCmd_flg(74)/1
  Demux/87 -> GaCBC_CellBalCtlCmd_flg(75)/1
  Demux/88 -> GaCBC_CellBalCtlCmd_flg(76)/1
  Demux/89 -> GaCBC_CellBalCtlCmd_flg(77)/1
  Demux/90 -> GaCBC_CellBalCtlCmd_flg(78)/1
  Demux/91 -> GaCBC_CellBalCtlCmd_flg(79)/1
  Demux/92 -> GaCBC_CellBalCtlCmd_flg(80)/1
  Demux/93 -> GaCBC_CellBalCtlCmd_flg(81)/1
  Demux/94 -> GaCBC_CellBalCtlCmd_flg(82)/1
  Demux/95 -> GaCBC_CellBalCtlCmd_flg(83)/1
  Demux/96 -> GaCBC_CellBalCtlCmd_flg(84)/1
  Demux/97 -> GaCBC_CellBalCtlCmd_flg(85)/1
  Demux/98 -> GaCBC_CellBalCtlCmd_flg(86)/1
  Demux/99 -> GaCBC_CellBalCtlCmd_flg(87)/1
  Demux/100 -> GaCBC_CellBalCtlCmd_flg(88)/1
  Demux/101 -> GaCBC_CellBalCtlCmd_flg(89)/1
  Demux/102 -> GaCBC_CellBalCtlCmd_flg(90)/1
  Demux/103 -> GaCBC_CellBalCtlCmd_flg(91)/1
  Demux/104 -> GaCBC_CellBalCtlCmd_flg(92)/1
  Demux/105 -> GaCBC_CellBalCtlCmd_flg(93)/1
  Demux/106 -> GaCBC_CellBalCtlCmd_flg(94)/1
  Demux/107 -> GaCBC_CellBalCtlCmd_flg(95)/1
  Demux/108 -> GaCBC_CellBalCtlCmd_flg(96)/1
  Demux/109 -> GaCBC_CellBalCtlCmd_flg(97)/1
  Demux/110 -> GaCBC_CellBalCtlCmd_flg(98)/1
  Demux/111 -> GaCBC_CellBalCtlCmd_flg(99)/1
  Demux/112 -> GaCBC_CellBalCtlCmd_flg(100)/1
  Demux/113 -> GaCBC_CellBalCtlCmd_flg(101)/1
  Demux/114 -> GaCBC_CellBalCtlCmd_flg(102)/1
  Demux/115 -> GaCBC_CellBalCtlCmd_flg(103)/1
  Demux/116 -> GaCBC_CellBalCtlCmd_flg(104)/1
  Demux/117 -> GaCBC_CellBalCtlCmd_flg(105)/1
  Demux/118 -> GaCBC_CellBalCtlCmd_flg(106)/1
  Demux/119 -> GaCBC_CellBalCtlCmd_flg(107)/1
  Demux/120 -> GaCBC_CellBalCtlCmd_flg(108)/1
  Demux/121 -> GaCBC_CellBalCtlCmd_flg(109)/1
  Demux/122 -> GaCBC_CellBalCtlCmd_flg(110)/1
  Demux/123 -> GaCBC_CellBalCtlCmd_flg(111)/1
  Demux/124 -> GaCBC_CellBalCtlCmd_flg(112)/1
  Demux/125 -> GcSOC_MaxCellSOC_pct/1
  Demux/126 -> GcSOC_MinCellSOC_pct/1
  Demux/127 -> GcSOC_PackSOC_pct/1
  Demux/128 -> GcSOH_PackSOH_pct/1
  Demux/129 -> GbISP_TFPosCtlLoadOpenFlt_flg/1
  Demux/130 -> GbISP_TFDCPosCtlLoadOpenFlt_flg/1
  Demux/131 -> GbISP_TFPreChrgFail_flg/1
  Demux/132 -> GbISP_TFPreChrgShrt_flg/1
  Demux/133 -> GbISP_TFPosCloseFlt_flg/1
  Demux/134 -> GbISP_TFPosOpenFlt_flg/1
  Demux/135 -> GbISP_TFNegCloseFlt_flg/1
  Demux/136 -> GbISP_TFNegOpenFlt_flg/1
  Demux/137 -> GbISP_TFBMUSpyStTooLow_flg/1
  Demux/138 -> GbISP_TFKL30CStTooLow_flg/1
  Demux/139 -> GeCTC_CtrCtlConnMode_enum/1
  Demux/140 -> GbISP_TFPreOpenFlt_flg/1
  Demux/141 -> GbISP_TFDCNegOpenFlt_flg/1
  Demux/142 -> GbISP_TFThmRnwyWarn_flg/1
  Demux/143 -> GbISP_TFThmRnwyAlrm_flg/1
  Demux/144 -> GbISP_TFThmRnwyfDet_flg/1
  Demux/145 -> GbWSM_TplWkUpPrs_flg/1
  Demux/146 -> GbISP_TFHvilLFlt_flg/1
  Demux/147 -> GbISP_TFHvilSTG_flg/1
  Demux/148 -> GbISP_TFHvilSTV_flg/1
  Demux/149 -> GbISP_TFIsoHVoffResFltLevel1_flg/1
  Demux/150 -> GbISP_TFIsoHVoffResFltLevel2_flg/1
  Demux/151 -> GbISP_TFIsoResFltLevel1_flg/1
  Demux/152 -> GbISP_TFIsoResFltLevel2_flg/1
  Demux/153 -> GbISP_TFIsoDCResFltLevel1_flg/1
  Demux/154 -> GbISP_TFIsoDCResFltLevel2_flg/1
  Demux/155 -> GbISP_TFCANCrashFlt_flg/1
  Demux/156 -> GbISP_TFHWCrashFlt_flg/1
